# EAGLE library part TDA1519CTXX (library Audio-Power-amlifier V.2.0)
22WBTL or 2 ´ 11Wstereo power amplifier
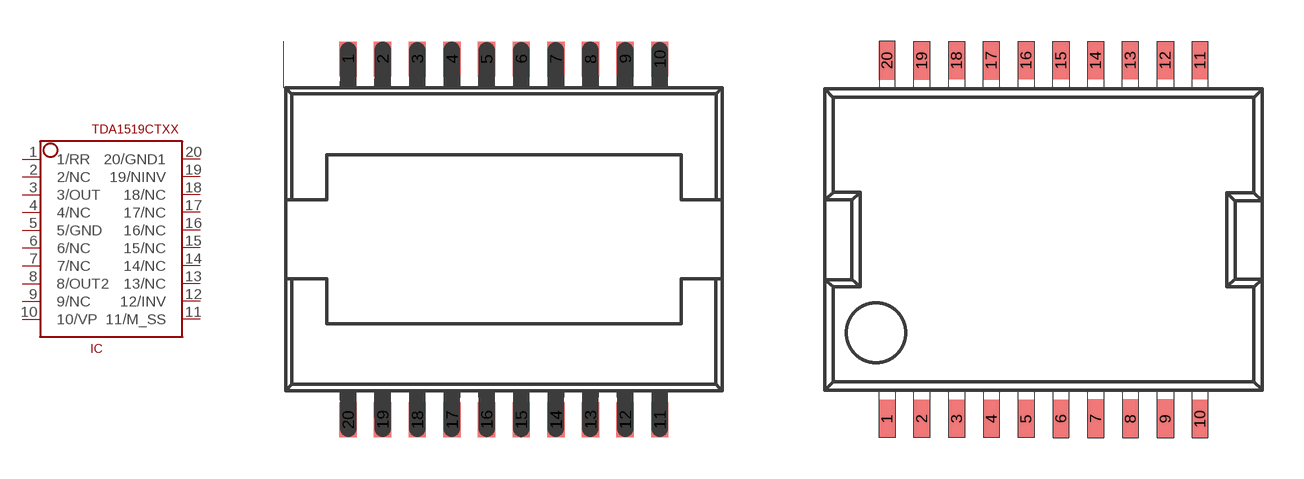
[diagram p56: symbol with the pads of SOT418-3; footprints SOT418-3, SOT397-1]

Designator prefix IC

## TDA1519CTXXTDA1519CTD  [SOT418-3]
1  1/RR
2  2/NC  nc
3  3/OUT  out
4  4/NC  nc
5  5/GND  pwr
6  6/NC  nc
7  7/NC  nc
8  8/OUT2  out
9  9/NC  nc
10  10/VP  pwr
11  11/M_SS
12  12/INV
13  13/NC  nc
14  14/NC  nc
15  15/NC  nc
16  16/NC  nc
17  17/NC  nc
18  18/NC  nc
19  19/NINV
20  20/GND1  pwr

## TDA1519CTXXTDA1519CTH  [SOT397-1]
Pads as for SOT418-3

## Footprint SOT418-3 (pad centres in mm)
smd 0.635 x 1.27: 1 -5.715,6.615; 2 -4.445,6.615; 3 -3.175,6.615; 4 -1.905,6.615; 5 -0.635,6.615; 6 0.635,6.615; 7 1.905,6.615; 8 3.175,6.615; 9 4.445,6.615; 10 5.715,6.615; 11 5.715,-6.615; 12 4.445,-6.615; 13 3.175,-6.615; 14 1.905,-6.615; 15 0.635,-6.615; 16 -0.635,-6.615; 17 -1.905,-6.615; 18 -3.175,-6.615; 19 -4.445,-6.615; 20 -5.715,-6.615

## Footprint SOT397-1 (pad centres in mm)
smd 0.6 x 1.4: 1 -5.715,-6.55; 2 -4.445,-6.55; 3 -3.17,-6.55; 4 -1.9,-6.55; 5 -0.635,-6.55; 6 0.64,-6.55; 7 1.91,-6.545; 8 3.18,-6.545; 9 4.455,-6.545; 10 5.72,-6.55; 11 5.72,6.55; 12 4.45,6.55; 13 3.175,6.55; 14 1.905,6.55; 15 0.64,6.55; 16 -0.635,6.55; 17 -1.905,6.545; 18 -3.175,6.55; 19 -4.445,6.545; 20 -5.715,6.545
